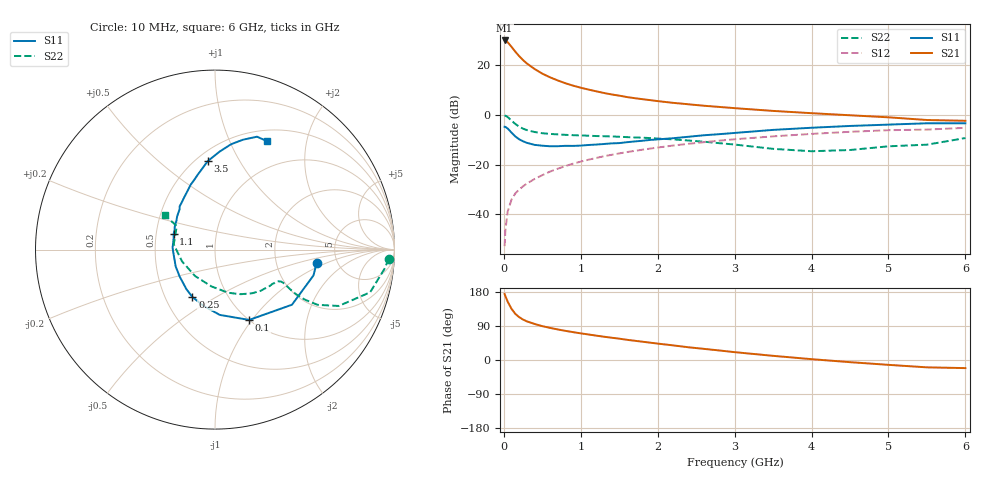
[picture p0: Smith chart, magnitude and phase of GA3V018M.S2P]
! Infineon Technologies  Discrete & RF Semiconductors
! BF775
! Si NPN RF Bipolar Junction Transistor in SOT23
! VCE = 3 V  IC = 18 mA
! Common Emitter S-Parameters:  May  1996
# GHz  S  MA  R  50
!  f  S11  S21  S12  S22
! GHz  MAG  ANG  MAG  ANG  MAG  ANG  MAG  ANG
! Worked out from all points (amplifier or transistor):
!   36 points, 10 MHz to 6 GHz, reference 50 ohm
!   highest |S21| = 29.8 dB at 10 MHz (marker M1)
!   |S21| within 3 dB of that: start of sweep to 111.1 MHz
!   unconditionally stable (mu >= 1): 398.7 MHz to 3.208 GHz
!   at 250 MHz: K = 0.85, MSG = 25.3 dB, |S12| = -28.7 dB
!   at 1.4 GHz: K = 1.12, MAG = 10.0 dB, |S12| = -16.1 dB
!   at 6 GHz: K = 0.96, MSG = 1.4 dB, |S12| = -5.3 dB
!   S11 on the Smith chart (normalised r, x): 10 MHz: 3.47, -0.78; 100 MHz: 1.00, -0.97; 250 MHz: 0.68, -0.39; 1.1 GHz: 0.62, +0.11; 3.5 GHz: 0.57, +0.74; 6 GHz: 0.63, +1.38
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0.01  0.5712 -7.6  30.78 174.3  0.0023 88.0  0.97 -3.0
0.02  0.5672 -14.7  30.38 168.6  0.0048 85.5  0.9508 -6.4
0.05  0.5275 -35.6  28.32 153.9  0.0114 75.3  0.8964 -15.4
0.1  0.4357 -64.1  22.91 134.9  0.0198 69.1  0.7574 -24.5
0.15  0.3648 -85.8  18.26 121.5  0.0264 65.0  0.6492 -28.3
0.2  0.3199 -101.6  14.91 113.0  0.0315 65.3  0.5738 -29.1
0.25  0.2926 -115.5  12.42 106.7  0.0366 65.3  0.5225 -28.9
0.3  0.272 -125.8  10.62 101.9  0.0415 66.7  0.4897 -28.3
0.4  0.2475 -142.9  8.226 95.1  0.0513 68.0  0.4482 -26.9
0.5  0.2383 -156.8  6.646 89.3  0.0611 69.0  0.4245 -26.0
0.6  0.2324 -166.1  5.612 84.8  0.072 69.3  0.4108 -25.8
0.8  0.2368 177.1  4.266 76.9  0.0928 68.8  0.3936 -26.6
0.9  0.2361 170.5  3.819 73.5  0.104 68.5  0.3874 -27.3
1.1  0.2462 159.8  3.185 67.4  0.1248 67.1  0.3781 -29.8
1.3  0.2577 150.6  2.722 61.5  0.1462 65.4  0.3691 -32.4
1.6  0.2801 138.9  2.255 53.3  0.1775 62.5  0.3543 -37.3
2.2  0.3366 120.9  1.724 38.6  0.2399 55.8  0.3194 -49.6
3  0.4295 102.8  1.35 20.7  0.3205 45.7  0.2513 -73.0
3.5  0.4945 94.7  1.188 11.0  0.3666 39.1  0.206 -95.6
4.5  0.5932 81.4  0.972 -5.7  0.4529 25.5  0.1952 -160.4
5.5  0.671 69.6  0.781 -19.4  0.5015 10.6  0.2499 148.4
6  0.6701 64.6  0.753 -21.4  0.5443 6.5  0.3394 145.6
